(* Logix 5000 AddOnInstructionDefinition export FormatEfloData; software revision 34.01 *)

TYPE EfloInputData :
STRUCT
   BC_FLOW : INT;   // Linearized flow
   BC_MA_IN : INT;   // Milliamp input from flow sensor
   BC_SETPOINT : INT;   // Setpoint
   BC_FLOW_DP : INT;   // Linearized flow decimal place
   BC_INST_ADDR : INT;   // modbus address
   BC_FULL_SCALE : INT;   // Full scale capacity
   BC_INLET_PRESSURE : INT;   // Inlet Pressure
   BC_DIFF_PRESSURE : INT;   // Differential pressure across the orifice
   BC_TEMPERATURE : INT;   // Temperature (1 decimal place)
   BC_MOTOR_POSITION : INT;   // 1 = 0.0032mm
   DUMMY_REG_1 : INT;   // Doesn't do anything.
   DUMMY_REG_2 : INT;   // Doesn't do anything.
   BC_AIR_FLOW : INT;   // Air Flow
   DUMMY_REG_3 : INT;   // Doesn't do anything.
   BC_DEVIATION_ALARM : INT;   // R/W, 0-9999 and will display flow decimal place
   BC_LOW_PRES_ALARM_VALUE : INT;   // R/W, to disable 0
   BC_LOW_FLOW_ALARM_VALUE : INT;   // R/W, to disable 0
   BC_HIGH_FLOW_ALARM_VALUE : INT;   // R/W, to disable 0
   BC_ALARM_BYTE : INT;   // Alarm bit map; bit 0 = HI Limit sw, low byte note used
   BC_AUTO_MAN : INT;   // 1 = auto, 0 = manual
   BC_TOT_UP_FLAG : INT;   // Update totalizer flag, low byte unused
   BC_TOTAL_RESET : INT;   // reset flow totalizer
   BC_TOTAL_REM : INT;   // Remainder of summer not > 3600
   BC_TOTAL_UNITS : INT;   // Totalizer accumulator units
   BC_TOTAL_10K : INT;   // Totalizer accumulator 10K
   BC_TOTAL_100M : INT;   // Totalizer accumulator 100M
END_STRUCT
END_TYPE

TYPE EfloOutputData :
STRUCT
   BC_SETPOINT : INT;   // Setpoint
   CONTROL_MODE_MB : INT;   // currently always zero
   BC_AUTO_MAN : INT;   // 1 = auto, 0 = manual
END_STRUCT
END_TYPE

ADD_ON_INSTRUCTION FormatEfloData   (* revision 1.0, vendor Super Systems, Inc. *)
VAR_IN_OUT
   InputBuffer : SINT[52]; {required}
   InputFormatted : EfloInputData; {required}
   OutputBuffer : SINT[6]; {required}
   OutputFormatted : EfloOutputData; {required}
END_VAR

ROUTINE Logic   (* ladder *)
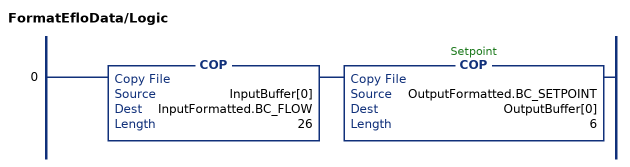
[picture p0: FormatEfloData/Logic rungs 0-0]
   0: COP(InputBuffer[0],InputFormatted.BC_FLOW,26)COP(OutputFormatted.BC_SETPOINT,OutputBuffer[0],6);
END_ROUTINE
END_ADD_ON_INSTRUCTION
